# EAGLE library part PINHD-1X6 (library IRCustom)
PIN HEADER
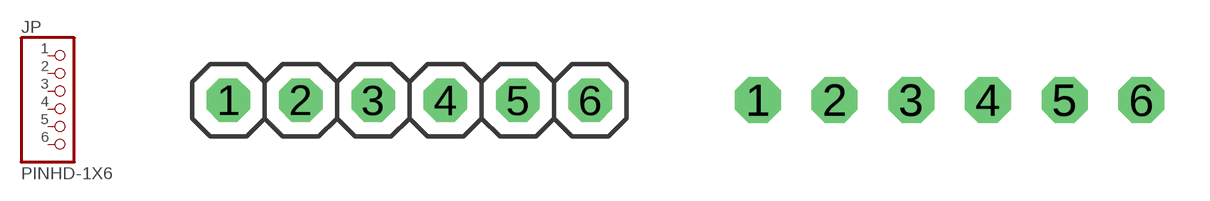
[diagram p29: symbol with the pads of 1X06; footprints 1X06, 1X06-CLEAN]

Designator prefix JP

## PINHD-1X6  [1X06]
1  1  pas
2  2  pas
3  3  pas
4  4  pas
5  5  pas
6  6  pas

## PINHD-1X6CLEAN  [1X06-CLEAN]
Pads as for 1X06

## PINHD-1X6CB  [1X06-CLEANBIG]
Pads as for 1X06

## PINHD-1X6B  [1X06-BIG]
Pads as for 1X06

## PINHD-1X6LOCK  [1X06-BIGLOCK]
Pads as for 1X06

## PINHD-1X6-3.5MM  [1X06-3.5MM]
Pads as for 1X06

## Footprint 1X06 (pad centres in mm)
PIN HEADER
drill 1.016 octagon: 1 -6.35,0; 2 -3.81,0; 3 -1.27,0; 4 1.27,0; 5 3.81,0; 6 6.35,0

## Footprint 1X06-CLEAN (pad centres in mm)
drill 1.016 octagon: 1 -6.35,0; 2 -3.81,0; 3 -1.27,0; 4 1.27,0; 5 3.81,0; 6 6.35,0

## Footprint 1X06-CLEANBIG (pad centres in mm)
drill 1.016 pad 1.778 octagon: 1 -6.35,0; 2 -3.81,0; 3 -1.27,0; 4 1.27,0; 5 3.81,0; 6 6.35,0

## Footprint 1X06-BIG (pad centres in mm)
drill 1.016 pad 1.778 octagon: 1 -6.35,0; 2 -3.81,0; 3 -1.27,0; 4 1.27,0; 5 3.81,0; 6 6.35,0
